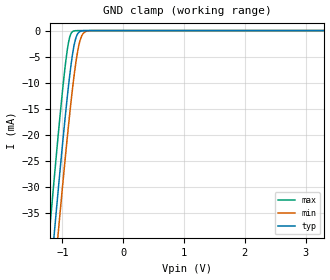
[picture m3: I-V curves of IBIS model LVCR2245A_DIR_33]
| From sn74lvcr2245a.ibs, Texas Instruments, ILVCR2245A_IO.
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[Model]   LVCR2245A_DIR_33
Model_type  Input
Vinl=0.8
Vinh=2.0
| variable   typ   min   max
C_comp   3.56pF   3.09pF   4.87pF
[Temperature Range]   40   100   -40
| Ambient temperature   25   85   -40
[Voltage range]   3.3   3   3.6
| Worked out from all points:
|   GND clamp passes 1 mA (typ) near -0.77 V on its own axis
[GND Clamp]
| LVCR2245A_DIR_33
|   Voltage   I(typ)   I(min)   I(max)
-5.5V     -655.9mA   -662.8mA   -647.2mA
-1.225V   -50.97mA   -59.27mA   -40.34mA
-1.145V   -40.41mA   -48.71mA   -29.75mA
-1.12V    -37.16mA   -45.45mA   -26.51mA
-1.08V    -32.01mA   -40.28mA   -21.4mA
-1.06V    -29.47mA   -37.73mA   -18.9mA
-965mV    -17.86mA   -25.89mA   -7.898mA
-885mV    -9.107mA   -16.56mA   -1.487mA
-780mV    -1.473mA   -6.233mA   -17.16uA
-715mV    -205.6uA   -2.13mA    -809.3nA
-640mV    -15.54uA   -338.4uA   -23.72nA
3.3V      6.304pA    9.26pA     5.93pA
